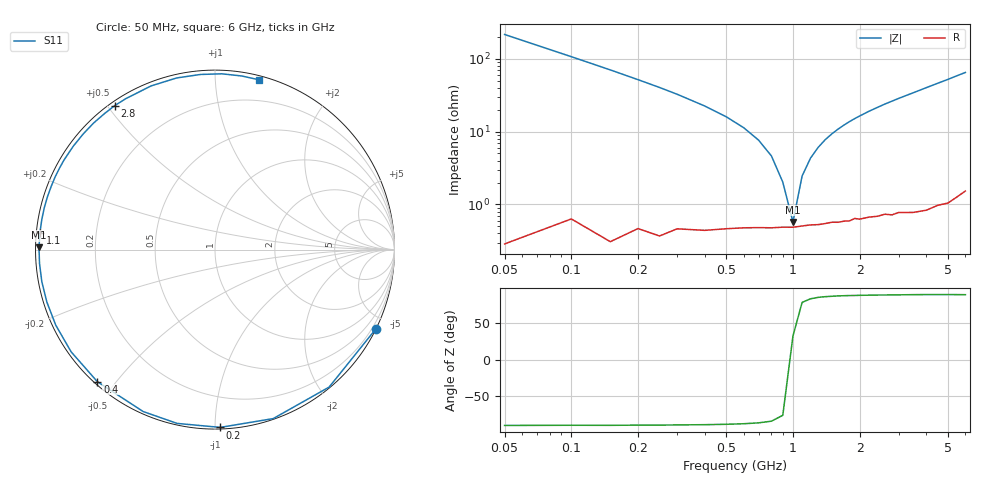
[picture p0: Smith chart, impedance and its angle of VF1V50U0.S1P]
! Infineon Technologies  Discrete & RF Semiconductors
! BBY 58-03
! Si Tuning Diode in SOD323
! VR = 1.5 V
! S-Parameters:  June  1999
# GHz  S  MA  R  50
!  f  S11
! GHz  MAG  ANG
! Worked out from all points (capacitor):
!   34 points, 50 MHz to 6 GHz, reference 50 ohm
!   read as one part to ground: C = 14.8 pF near 50 MHz
!   lowest |Z| = 575 mohm at 1 GHz (marker M1)
!   series resonance near 986.5 MHz, so ESL is about 1.8 nH
!   S11 on the Smith chart (normalised r, x): 50 MHz: 0.01, -4.30; 200 MHz: 0.01, -1.03; 400 MHz: 0.01, -0.45; 1.1 GHz: 0.01, +0.05; 2.8 GHz: 0.01, +0.52; 6 GHz: 0.03, +1.29
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0.05  0.9994 -26.2
0.1  0.9954 -50.3
0.15  0.9959 -71.0
0.2  0.991 -88.3
0.25  0.9911 -102.3
0.3  0.9871 -113.9
0.4  0.9854 -131.7
0.5  0.9833 -144.6
0.6  0.982 -154.6
0.7  0.9814 -162.7
0.8  0.9812 -169.5
0.9  0.9807 -175.5
1  0.9807 179.3
1.1  0.98 174.5
1.4  0.9788 162.4
1.6  0.9785 155.6
1.8  0.9781 149.4
2  0.9775 143.8
2.2  0.9769 138.5
2.4  0.977 133.7
2.8  0.9776 124.8
3  0.9769 120.6
3.5  0.979 111.3
4  0.9799 102.6
4.5  0.9791 94.8
5  0.9801 87.8
5.5  0.9788 81.2
6  0.9774 75.4
